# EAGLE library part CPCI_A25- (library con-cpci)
Compact PCI A 25 Source: www.erni.com
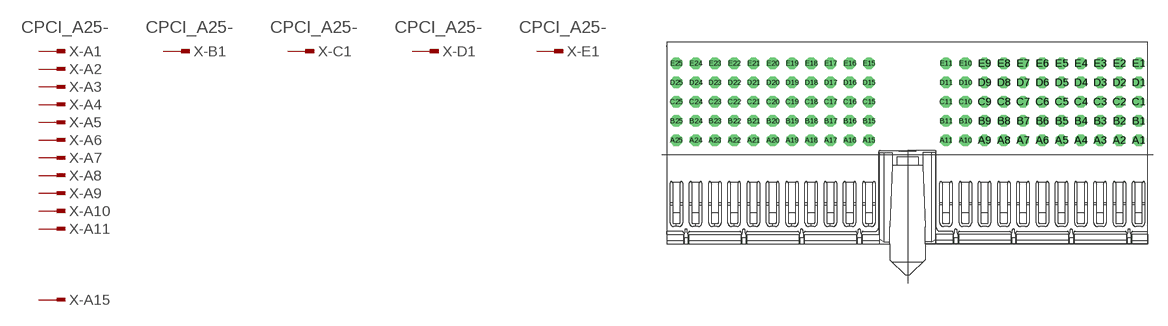
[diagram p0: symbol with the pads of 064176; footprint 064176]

Designator prefix X; gates -A1=PINV -B1=PINV -C1=PINV -D1=PINV -E1=PINV -A2=PIN -A3=PIN -A4=PIN -A5=PIN -A6=PIN -A7=PIN -A8=PIN -A9=PIN -A10=PIN -A11=PIN -A15=PIN -A16=PIN -A17=PIN -A18=PIN -A19=PIN -A20=PIN -A21=PIN -A22=PIN -A23=PIN -A24=PIN -A25=PIN -B2=PIN -B3=PIN -B4=PIN -B5=PIN -B6=PIN -B7=PIN -B8=PIN -B9=PIN -B10=PIN -B11=PIN -B15=PIN -B16=PIN -B17=PIN -B18=PIN -B19=PIN -B20=PIN -B21=PIN -B22=PIN -B23=PIN -B24=PIN -B25=PIN -C2=PIN -C3=PIN -C4=PIN -C5=PIN -C6=PIN -C7=PIN -C8=PIN -C9=PIN -C10=PIN -C11=PIN -C15=PIN -C16=PIN -C17=PIN -C18=PIN -C19=PIN -C20=PIN -C21=PIN -C22=PIN -C23=PIN -C24=PIN -C25=PIN -D2=PIN -D3=PIN -D4=PIN -D5=PIN -D6=PIN -D7=PIN -D8=PIN -D9=PIN -D10=PIN -D11=PIN -D15=PIN -D16=PIN -D17=PIN -D18=PIN -D19=PIN -D20=PIN -D21=PIN -D22=PIN -D23=PIN -D24=PIN -D25=PIN -E2=PIN -E3=PIN -E4=PIN -E5=PIN -E6=PIN -E7=PIN -E8=PIN -E9=PIN -E10=PIN -E11=PIN -E15=PIN -E16=PIN -E17=PIN -E18=PIN -E19=PIN -E20=PIN -E21=PIN -E22=PIN -E23=PIN -E24=PIN -E25=PIN

## CPCI_A25-064176 (OC_FARNELL: unknown; OC_NEWARK: unknown)  [064176]
A1  -A1:1  in
A2  -A2:1  in
A3  -A3:1  in
A4  -A4:1  in
A5  -A5:1  in
A6  -A6:1  in
A7  -A7:1  in
A8  -A8:1  in
A9  -A9:1  in
A10  -A10:1  in
A11  -A11:1  in
A15  -A15:1  in
A16  -A16:1  in
A17  -A17:1  in
A18  -A18:1  in
A19  -A19:1  in
A20  -A20:1  in
A21  -A21:1  in
A22  -A22:1  in
A23  -A23:1  in
A24  -A24:1  in
A25  -A25:1  in
B1  -B1:1  in
B2  -B2:1  in
B3  -B3:1  in
B4  -B4:1  in
B5  -B5:1  in
B6  -B6:1  in
B7  -B7:1  in
B8  -B8:1  in
B9  -B9:1  in
B10  -B10:1  in
B11  -B11:1  in
B15  -B15:1  in
B16  -B16:1  in
B17  -B17:1  in
B18  -B18:1  in
B19  -B19:1  in
B20  -B20:1  in
B21  -B21:1  in
B22  -B22:1  in
B23  -B23:1  in
B24  -B24:1  in
B25  -B25:1  in
C1  -C1:1  in
C2  -C2:1  in
C3  -C3:1  in
C4  -C4:1  in
C5  -C5:1  in
C6  -C6:1  in
C7  -C7:1  in
C8  -C8:1  in
C9  -C9:1  in
C10  -C10:1  in
C11  -C11:1  in
C15  -C15:1  in
C16  -C16:1  in
C17  -C17:1  in
C18  -C18:1  in
C19  -C19:1  in
C20  -C20:1  in
C21  -C21:1  in
C22  -C22:1  in
C23  -C23:1  in
C24  -C24:1  in
C25  -C25:1  in
D1  -D1:1  in
D2  -D2:1  in
D3  -D3:1  in
D4  -D4:1  in
D5  -D5:1  in
D6  -D6:1  in
D7  -D7:1  in
D8  -D8:1  in
D9  -D9:1  in
D10  -D10:1  in
D11  -D11:1  in
D15  -D15:1  in
D16  -D16:1  in
D17  -D17:1  in
D18  -D18:1  in
D19  -D19:1  in
D20  -D20:1  in
D21  -D21:1  in
D22  -D22:1  in
D23  -D23:1  in
D24  -D24:1  in
D25  -D25:1  in
E1  -E1:1  in
E2  -E2:1  in
E3  -E3:1  in
E4  -E4:1  in
E5  -E5:1  in
E6  -E6:1  in
E7  -E7:1  in
E8  -E8:1  in
E9  -E9:1  in
E10  -E10:1  in
E11  -E11:1  in
E15  -E15:1  in
E16  -E16:1  in
E17  -E17:1  in
E18  -E18:1  in
E19  -E19:1  in
E20  -E20:1  in
E21  -E21:1  in
E22  -E22:1  in
E23  -E23:1  in
E24  -E24:1  in
E25  -E25:1  in

## Footprint 064176 (pad centres in mm)
ERmet Federleiste A / ERmet Female Type A ohne Fixierstift / without locating pegs Abschirmblech oben montiert / shielding mounted on top Source: http://www.erni.com/DB/PDF-Drawing/ERmet/064176.pdf
drill 0.7 pad 1.016 octagon: A1 24,0; A2 22,0; A3 20,0; A4 18,0; A5 16,0; A6 14,0; A7 12,0; A8 10,0; A9 8,0; A10 6,0; A11 4,0; A15 -4,0; A16 -6,0; A17 -8,0; A18 -10,0; A19 -12,0; A20 -14,0; A21 -16,0; A22 -18,0; A23 -20,0; A24 -22,0; A25 -24,0; B1 24,2; B2 22,2; B3 20,2; B4 18,2; B5 16,2; B6 14,2; B7 12,2; B8 10,2; B9 8,2; B10 6,2; B11 4,2; B15 -4,2; B16 -6,2; B17 -8,2; B18 -10,2; B19 -12,2; B20 -14,2; B21 -16,2; B22 -18,2; B23 -20,2; B24 -22,2; B25 -24,2; C1 24,4; C2 22,4; C3 20,4; C4 18,4; C5 16,4; C6 14,4; C7 12,4; C8 10,4; C9 8,4; C10 6,4; C11 4,4; C15 -4,4; C16 -6,4; C17 -8,4; C18 -10,4; C19 -12,4; C20 -14,4; C21 -16,4; C22 -18,4; C23 -20,4; C24 -22,4; C25 -24,4; D1 24,6; D2 22,6; D3 20,6; D4 18,6; D5 16,6; D6 14,6; D7 12,6; D8 10,6; D9 8,6; D10 6,6; D11 4,6; D15 -4,6; D16 -6,6; D17 -8,6; D18 -10,6; D19 -12,6; D20 -14,6; D21 -16,6; D22 -18,6; D23 -20,6; D24 -22,6; D25 -24,6; E1 24,8; E2 22,8; E3 20,8; E4 18,8; E5 16,8; E6 14,8; E7 12,8; E8 10,8; E9 8,8; E10 6,8; E11 4,8; E15 -4,8; E16 -6,8; E17 -8,8; E18 -10,8; E19 -12,8; E20 -14,8; E21 -16,8; E22 -18,8; E23 -20,8; E24 -22,8; E25 -24,8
